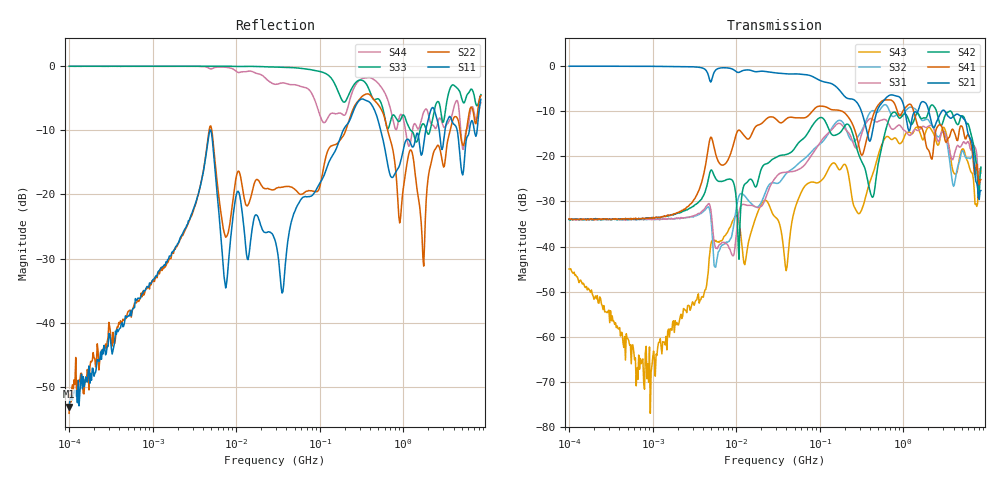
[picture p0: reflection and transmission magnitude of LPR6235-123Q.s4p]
# MHz S MA R 50
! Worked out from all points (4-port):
!   498 points, 100 kHz to 8.5 GHz, reference 50 ohm
!   strongest paths, dB at 100 kHz, 1.698 MHz, 29.49 MHz, 500.7 MHz, 8.5 GHz:
!     S21: -0.1, -0.1, -1.5, -9.4, -27.6
!     S41: -33.9, -33.0, -11.7, -8.7, -25.2
!     S42: -33.9, -32.9, -20.3, -21.8, -22.4
!     S31: -33.9, -33.8, -24.8, -12.3, -22.5
!     S32: -34.0, -33.9, -26.0, -10.2, -23.7
!     S43: -45.0, -58.5, -33.5, -19.8, -23.3
!   lowest |S11| = -53.0 dB at 100 kHz (marker M1), VSWR 1.00, Z = 50.2 + j0.128 ohm
!   |S11| at or under -10 dB: 536.3 MHz to 1.861 GHz (1.325 GHz wide, 111 % of centre); 4.415 GHz to 6.197 GHz (1.782 GHz wide, 33.6 % of centre); 7.079 GHz to 7.658 GHz (578.2 MHz wide, 7.85 % of centre)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
0.1  0.002248 34.7  0.9934 -0.2  0.02008 -179.4  0.02024 4.0
     0.9934 -0.2  0.001991 69.9  0.01987 1.4  0.02009 178.8
     0.02008 -179.4  0.01987 1.4  0.9924 0.3  0.005636 -86.1
     0.02024 4.0  0.02009 178.8  0.005636 -86.1  0.9928 0.2
0.8956976  0.01899 72.6  0.9908 -1.7  0.01997 174.8  0.02059 21.9
           0.9908 -1.7  0.01927 82.2  0.02028 0.9  0.02078 155.0
           0.01997 174.8  0.02028 0.9  0.9926 -0.2  0.0003144 18.6
           0.02059 21.9  0.02078 155.0  0.0003144 18.6  0.9921 -1.0
9.853441  0.09429 -15.9  0.8753 -10.0  0.01172 -163.4  0.1666 71.0
          0.8753 -10.0  0.1292 43.5  0.02381 83.7  0.03909 23.3
          0.01172 -163.4  0.02381 83.7  0.99 -3.5  0.02205 50.8
          0.1666 71.0  0.03909 23.3  0.02205 50.8  0.9147 -13.4
1039.755  0.2479 -86.0  0.329 -174.0  0.1926 -143.6  0.3373 -143.7
          0.329 -174.0  0.1323 -158.9  0.3022 -128.7  0.2951 -116.6
          0.1926 -143.6  0.3022 -128.7  0.404 -167.6  0.1687 -93.9
          0.3373 -143.7  0.2951 -116.6  0.1687 -93.9  0.3464 177.7
2713.323  0.3043 -14.3  0.2827 10.5  0.1514 -4.3  0.2237 9.2
          0.2827 10.5  0.2308 18.7  0.1662 -14.9  0.2352 -9.1
          0.1514 -4.3  0.1662 -14.9  0.5072 4.3  0.1445 22.4
          0.2237 9.2  0.2352 -9.1  0.1445 22.4  0.3922 -10.7
4284.188  0.3376 178.8  0.2904 154.3  0.1217 163.5  0.1616 160.5
          0.2904 154.3  0.4022 -159.5  0.06246 -175.4  0.2353 138.9
          0.1217 163.5  0.06246 -175.4  0.6848 -179.4  0.06384 177.0
          0.1616 160.5  0.2353 138.9  0.06384 177.0  0.5293 -171.7
8500  0.5486 -35.4  0.0417 4.2  0.07471 4.9  0.05506 -14.7
      0.0417 4.2  0.5852 -34.4  0.06529 34.9  0.0758 0.7
      0.07471 4.9  0.06529 34.9  0.5972 -46.2  0.06825 49.5
      0.05506 -14.7  0.0758 0.7  0.06825 49.5  0.5172 -38.1
